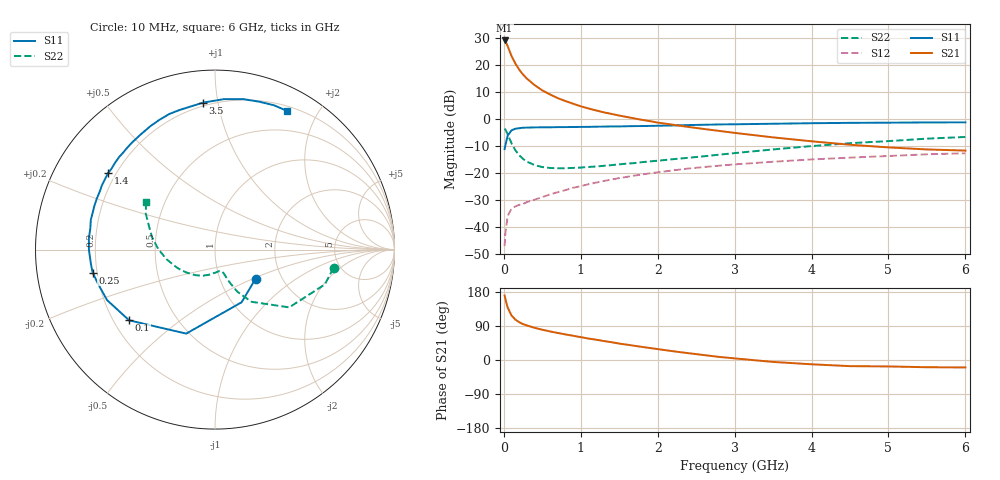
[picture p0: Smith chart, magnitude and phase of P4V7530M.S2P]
! SIEMENS Small Signal Semiconductors
! BFP182
! Si NPN RF Bipolar Junction Transistor in SOT143
! VCE = 0.75 V  IC = 30 mA
! Common Emitter S-Parameters:  March  1996
# GHz  S  MA  R  50
!  f  S11  S21  S12  S22
! GHz  MAG  ANG  MAG  ANG  MAG  ANG  MAG  ANG
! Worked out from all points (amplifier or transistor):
!   36 points, 10 MHz to 6 GHz, reference 50 ohm
!   highest |S21| = 29.2 dB at 10 MHz (marker M1)
!   |S21| within 3 dB of that: start of sweep to 61.95 MHz
!   unconditionally stable (mu >= 1): start of sweep to 28.22 MHz; 159.6 MHz to end of sweep
!   at 250 MHz: K = 1.36, MAG = 20.4 dB, |S12| = -31.5 dB
!   at 1.4 GHz: K = 2.39, MAG = 5.6 dB, |S12| = -22.4 dB
!   at 6 GHz: K = 1.89, MAG = -4.9 dB, |S12| = -12.7 dB
!   S11 on the Smith chart (normalised r, x): 10 MHz: 1.48, -0.52; 100 MHz: 0.26, -0.34; 250 MHz: 0.18, -0.09; 1.4 GHz: 0.17, +0.31; 3.5 GHz: 0.18, +0.91; 6 GHz: 0.25, +1.62
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0.01  0.2783 -35.6  28.81 170.3  0.0044 70.3  0.6685 -8.8
0.02  0.3288 -63.2  27.93 161.1  0.0076 69.8  0.6421 -17.6
0.05  0.4947 -108.9  22.54 138.3  0.016 54.2  0.5241 -37.9
0.1  0.6198 -140.5  14.83 117.4  0.0218 39.3  0.3551 -55.0
0.15  0.6639 -154.9  10.74 106.5  0.0241 35.9  0.2649 -62.1
0.2  0.6786 -163.5  8.281 99.7  0.0257 36.2  0.2138 -65.0
0.25  0.6939 -169.4  6.705 94.7  0.0267 37.8  0.1826 -67.1
0.3  0.6962 -173.8  5.645 91.1  0.0289 39.8  0.1625 -68.3
0.4  0.7025 179.9  4.272 84.9  0.032 42.4  0.1404 -69.9
0.5  0.7053 174.9  3.414 79.9  0.0359 45.2  0.1292 -71.9
0.6  0.7045 170.5  2.872 75.4  0.0401 48.6  0.1242 -74.7
0.7  0.7117 166.4  2.453 71.4  0.0441 49.9  0.1225 -77.5
0.9  0.715 160.0  1.933 64.0  0.0532 52.3  0.1245 -83.4
1.1  0.7188 153.4  1.577 56.6  0.062 53.1  0.1296 -90.4
1.4  0.7324 144.4  1.25 47.0  0.0759 52.8  0.1402 -101.0
1.8  0.7443 133.4  0.968 34.4  0.0941 50.5  0.1596 -114.1
2.2  0.763 123.1  0.787 23.1  0.112 46.7  0.1808 -128.2
2.8  0.7973 108.6  0.605 8.1  0.1371 40.3  0.2193 -148.5
3.5  0.8217 94.6  0.459 -5.1  0.1621 32.4  0.2742 -168.4
4.5  0.8533 79.2  0.335 -16.2  0.1932 21.6  0.3579 168.8
5.5  0.8686 67.9  0.274 -19.1  0.2227 11.3  0.4345 152.6
6  0.8709 62.5  0.261 -19.6  0.2327 5.6  0.4671 145.3
